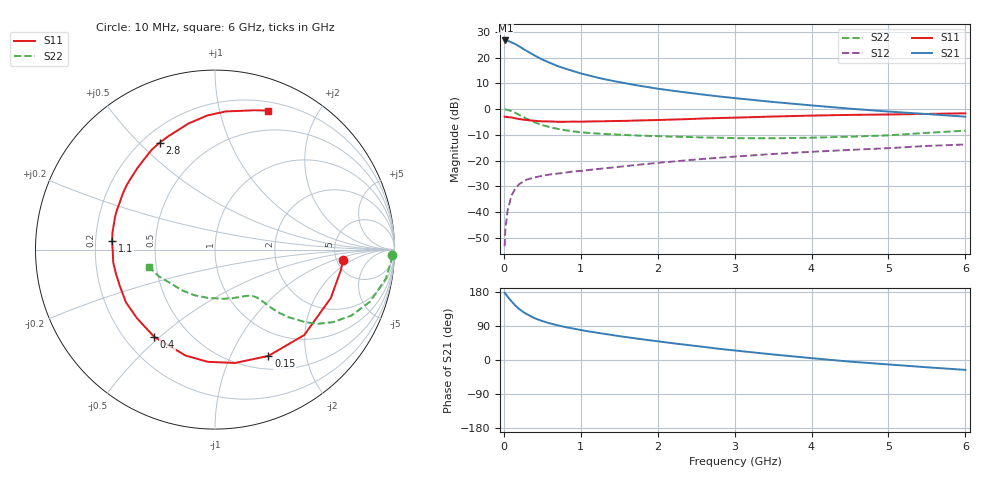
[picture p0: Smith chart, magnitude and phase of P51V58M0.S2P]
! SIEMENS Small Signal Semiconductors
! BFP183
! Si NPN RF Bipolar Junction Transistor in SOT143
! VCE = 1.5 V  IC = 8 mA
! Common Emitter S-Parameters:  March  1996
# GHz  S  MA  R  50
!  f  S11  S21  S12  S22
! GHz  MAG  ANG  MAG  ANG  MAG  ANG  MAG  ANG
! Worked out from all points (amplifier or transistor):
!   36 points, 10 MHz to 6 GHz, reference 50 ohm
!   highest |S21| = 26.6 dB at 20 MHz (marker M1)
!   |S21| within 3 dB of that: start of sweep to 236.4 MHz
!   unconditionally stable (mu >= 1): 1.221 GHz to 5.679 GHz
!   at 250 MHz: K = 0.29, MSG = 25.8 dB, |S12| = -28.2 dB
!   at 1.4 GHz: K = 1.07, MAG = 15.3 dB, |S12| = -22.7 dB
!   at 6 GHz: K = 0.96, MSG = 5.4 dB, |S12| = -13.7 dB
!   S11 on the Smith chart (normalised r, x): 10 MHz: 5.70, -1.34; 150 MHz: 0.66, -1.40; 400 MHz: 0.32, -0.48; 1.1 GHz: 0.27, +0.04; 2.8 GHz: 0.27, +0.58; 6 GHz: 0.29, +1.41
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0.01  0.7155 -4.6  21.3 177.5  0.0022 83.8  0.986 -1.9
0.02  0.7106 -9.3  21.43 175.1  0.0048 83.3  0.9832 -3.9
0.05  0.6994 -22.7  21.13 166.8  0.011 80.6  0.9658 -9.6
0.1  0.6885 -43.7  19.64 154.7  0.0212 69.0  0.9118 -18.5
0.15  0.6629 -63.3  18.18 143.6  0.0291 61.4  0.8442 -25.8
0.2  0.6414 -80.0  16.47 134.5  0.0351 55.2  0.7729 -31.5
0.25  0.6265 -93.6  14.71 127.0  0.0391 50.6  0.7066 -35.8
0.3  0.6129 -105.5  13.36 120.8  0.0431 47.1  0.6475 -38.7
0.4  0.5927 -124.8  10.97 110.3  0.0472 42.3  0.5545 -42.7
0.5  0.579 -138.7  9.121 102.8  0.051 39.1  0.4899 -45.0
0.6  0.5766 -149.4  7.885 96.7  0.054 37.7  0.4462 -46.1
0.7  0.5679 -158.5  6.828 91.5  0.0563 37.1  0.4132 -46.8
0.9  0.5715 -172.8  5.466 83.0  0.0617 37.0  0.3705 -48.1
1.1  0.5756 175.4  4.515 75.5  0.066 37.6  0.3454 -49.6
1.5  0.5895 157.8  3.336 63.0  0.0762 38.9  0.3185 -53.9
1.8  0.605 146.4  2.779 54.6  0.0849 39.1  0.3048 -58.6
2.2  0.627 133.6  2.266 44.1  0.0964 38.5  0.2924 -65.9
2.8  0.671 117.4  1.759 29.5  0.1141 36.2  0.2788 -79.6
3.5  0.7179 101.9  1.375 14.6  0.1349 32.8  0.272 -98.7
4.5  0.7723 85.5  1.02 -4.3  0.1619 26.1  0.2923 -129.2
5.5  0.8069 74.2  0.802 -19.2  0.1931 19.5  0.3463 -154.5
6  0.8287 69.2  0.714 -26.1  0.2062 15.2  0.3815 -165.7
